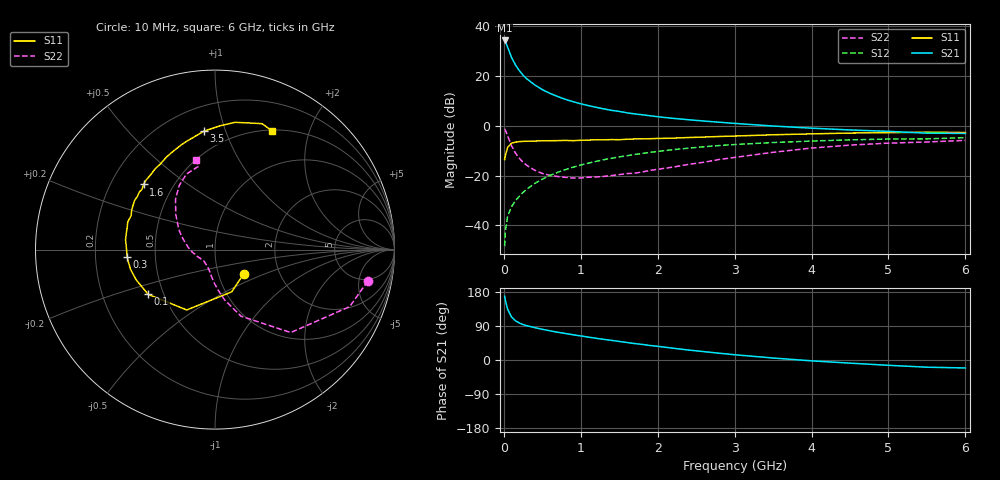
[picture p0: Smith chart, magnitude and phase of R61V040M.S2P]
! SIEMENS Small Signal Semiconductors
! BFR193
! Si NPN RF Bipolar Junction Transistor in SOT23
! VCE = 1 V  IC = 40 mA
! Common Emitter S-Parameters:  May  1996
# GHz  S  MA  R  50
!  f  S11  S21  S12  S22
! GHz  MAG  ANG  MAG  ANG  MAG  ANG  MAG  ANG
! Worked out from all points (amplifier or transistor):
!   36 points, 10 MHz to 6 GHz, reference 50 ohm
!   highest |S21| = 34.4 dB at 10 MHz (marker M1)
!   |S21| within 3 dB of that: start of sweep to 52.61 MHz
!   unconditionally stable (mu >= 1): 309.9 MHz to 2.281 GHz
!   at 250 MHz: K = 0.97, MSG = 23.6 dB, |S12| = -26.8 dB
!   at 1.4 GHz: K = 1.04, MAG = 8.5 dB, |S12| = -13.0 dB
!   at 6 GHz: K = 0.99, MSG = 0.9 dB, |S12| = -4.7 dB
!   S11 on the Smith chart (normalised r, x): 10 MHz: 1.32, -0.37; 100 MHz: 0.41, -0.26; 300 MHz: 0.34, -0.04; 1.6 GHz: 0.34, +0.35; 3.5 GHz: 0.36, +0.84; 6 GHz: 0.51, +1.46
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0.01  0.21 -40.2  52.34 168.2  0.0038 79.3  0.8691 -11.6
0.02  0.2531 -68.6  49.59 157.3  0.0077 72.7  0.8154 -22.9
0.05  0.3714 -115.1  37.96 133.4  0.0155 65.8  0.6259 -47.6
0.1  0.4483 -146.2  23.93 113.6  0.0236 63.6  0.3986 -68.6
0.15  0.4707 -159.2  16.95 103.7  0.0311 65.7  0.2858 -79.2
0.2  0.4828 -166.6  13.01 97.8  0.0382 68.6  0.2244 -85.8
0.25  0.4878 -171.9  10.47 93.5  0.0459 69.5  0.1846 -91.6
0.3  0.4913 -175.4  8.802 90.4  0.0535 71.4  0.16 -95.6
0.4  0.4947 177.9  6.698 85.5  0.0692 71.8  0.1285 -102.9
0.5  0.5015 173.7  5.366 81.0  0.0846 71.7  0.1103 -109.9
0.6  0.5026 169.2  4.497 77.0  0.1007 70.8  0.101 -116.4
0.7  0.505 165.4  3.895 73.2  0.1163 70.2  0.0959 -121.8
0.8  0.5102 162.4  3.423 69.9  0.132 69.0  0.0922 -127.4
1.1  0.5183 152.0  2.554 60.3  0.1783 65.0  0.0928 -141.1
1.3  0.5239 145.8  2.195 54.5  0.2087 62.0  0.0963 -150.8
1.6  0.5387 137.6  1.83 46.2  0.2513 57.2  0.1098 -162.8
2.2  0.5663 122.5  1.418 31.1  0.3324 47.2  0.1483 175.8
2.8  0.6118 108.2  1.185 17.9  0.4021 37.1  0.2108 155.4
3.5  0.6625 95.4  0.993 5.2  0.4621 25.4  0.2943 138.0
4.5  0.7176 81.1  0.828 -8.3  0.5234 11.3  0.4104 118.9
5.5  0.749 69.5  0.713 -19.0  0.5487 -2.0  0.4743 100.8
6  0.7341 64.4  0.706 -21.0  0.5799 -6.0  0.5109 102.1
